(* Logix 5000 AddOnInstructionDefinition export AMCI_MA_SD_SMD_Linear_Follower_CIPSYNC; software revision 20.05 *)

TYPE AMCI_Motion_Axis_Output_Data :
STRUCT
   Control_Word_0 : INT;
   Control_Word_1 : INT;
   Position_or_Distance : DINT;
   Programmed_Speed : DINT;
   Acceleration : INT;
   Deceleration : INT;
   Output_Word_8 : INT;
   Output_Word_9 : INT;
END_STRUCT
END_TYPE

TYPE AMCI_Motion_Axis_Input_Data :
STRUCT
   Moving_CW : BOOL;
   Moving_CCW : BOOL;
   In_Hold_State : BOOL;
   Stopped : BOOL;
   At_Home : BOOL;
   Accelerating : BOOL;
   Decelerating : BOOL;
   Move_Complete : BOOL;
   Status_Word_0_Bit_8 : BOOL;
   Status_Word_0_Bit_9 : BOOL;
   Position_Invalid : BOOL;
   Input_Error : BOOL;
   Command_Error : BOOL;
   Configuration_Error : BOOL;
   Module_OK : BOOL;
   Mode_Flag : BOOL;
   IN1_Active : BOOL;
   IN2_Active : BOOL;
   IN3_Active : BOOL;
   IN4_Active : BOOL;
   Status_Word_1_Bit_4 : BOOL;
   Status_Word_1_Bit_5 : BOOL;
   Connection_Was_Lost : BOOL;
   Driver_Fault : BOOL;
   Status_Word_1_Bit_8 : BOOL;
   Invalid_Jog_Change : BOOL;
   Status_Word_1_Bit_10 : BOOL;
   Heartbeat_Bit : BOOL;
   Status_Word_1_Bit_12 : BOOL;
   Status_Word_1_Bit_13 : BOOL;
   Stall_Detected : BOOL;
   Drive_Is_Enabled : BOOL;
   Motor_Position : DINT;
   Encoder_Position : DINT;
   Trapped_Encoder_Position : DINT;
   Input_Word_8 : INT;
   Input_Word_9 : INT;
END_STRUCT
END_TYPE

ADD_ON_INSTRUCTION AMCI_MA_SD_SMD_Linear_Follower_CIPSYNC   (* revision 1.0, vendor AMCI, ExecuteEnableInFalse *)
// Linear Axis Follower for SD and SMD devices.   Will not work with SV integrated servo devices.
// Revision note:
// 8/8/24.  Added timesync functionality to a previously existing AOI.  Also added logic to preset the motor position to the master axis position when the rung with the AOI becomes true, or if the master axis position changes when motion is not occurring.
// Help:
// MOTION AXIS SD & SMD LINEAR FOLLOWER
// These AOIs will only work with the SD and SMD motion devices.  The SV motion devices have their own follower AOIs.
// AXIS INPUT DATA:  Input data from AMCI motion device.   Uses the AMCI_Motion_Axis_Input_Data User Defined Data Type.
// AXIS OUTPUT DATA; Output data from the AOI to the AMCI motion device.   Uses the AMCI_Motion_Axis_Output_Data User Defined Data Type.
// FOLLOWER POSITION: REAL DATA TYPE position directly from the motion axis.
// FOLLOWER VELOCITY: REAL DATA TYPE velocity directly from the motion axis.
// ACCELERATION & DECELERATION: An actual value or an INT DATA TYPE.  Larger acceleration and
//                                                             deceleration values will cause the motion device to more quickly react
//                                                              changes in the source position and velocity values.
// PROPORTIONAL COEFFICIENT:  A value of 1 or 2 is recommended
// NETWORK DELAY: A value of zero, or 1 to the RPI time, will work in most applications.
// RPI_TIME: The RPI time used when adding the AMCI Motion device to the network.   8ms is the default.
//                    Used to control how long the preset motor command is sent to the device when the rung with the
//                    AOI transitions from false to true.
// TIMESYNC: The PLC's time value used to more closely synchronize the motion data from the PLC's master
//                     axis with the output of the AMCI motion device.
// EN (Enable) Set when rung is true, Reset when rung is false
// DN (Done) Set when command is sent to the motion device.  Reset when the rung is false.
// ER (Error) Set when a command or input error failed to clear.  Reset when the rung is false.
// IP (In Process) Set when follower command is active, even if motion is not occurring.   Reset when the rung
//                         goes false.
VAR_IN_OUT
   Axis_Input_Data : AMCI_Motion_Axis_Input_Data; {required}
   Axis_Output_Data : AMCI_Motion_Axis_Output_Data; {required}
END_VAR
VAR_INPUT
   Current_System_Time : DINT; {required}
   _0_for_Normal_1_for_Continuous : BOOL;
   Master_Axis_Position : REAL; {required}
   Master_Axis_Velocity : REAL; {required}
   Acceleration : INT; {required}
   Deceleration : INT; {required}
   Proportional_Coefficient : INT; {required}
   RPI_time_in_ms : DINT; {required}
END_VAR
VAR_OUTPUT
   EN : BOOL; {visible}
   ER : BOOL; {visible}
   DN : BOOL; {visible}
   IP : BOOL; {visible}
END_VAR
VAR
   command_data_block : INT[10];
        [0]   // Command Bits MSW
        [1]   // Command Bits LSW
        [2]   // Upper Target Position
        [3]   // Lower Target Position
        [4]   // Upper Programmed Speed
        [5]   // Lower Programmed Speed
   axis_follower_position : DINT;
   axis_follower_velocity : DINT;
   Preset_Motor_Position_timer_dynanic : TIMER; {access None}
   preset_one_shot : BOOL; {access None}
   RPI_div_1000 : REAL; {access None}
   difference_scan_position : DINT; {access None}
   last_scan_position : DINT; {access None}
   position_difference : DINT; {access None}
   position_last_scan_linear_SMD : DINT; {access None}
END_VAR

ROUTINE EnableInFalse   (* ladder *)
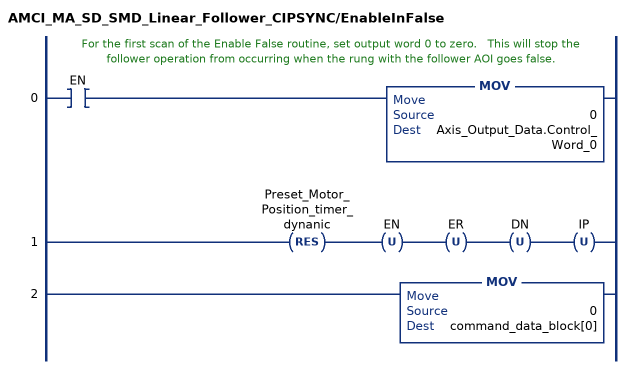
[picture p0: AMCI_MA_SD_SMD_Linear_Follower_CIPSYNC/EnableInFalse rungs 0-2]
   // For the first scan of the Enable False routine, set output word 0 to zero.   This will stop the follower operation from occurring when the rung with the follower AOI goes false.
   0: XIC(EN)MOV(0,Axis_Output_Data.Control_Word_0);
   1: RES(Preset_Motor_Position_timer_dynanic)OTU(EN)OTU(ER)OTU(DN)OTU(IP);
   2: MOV(0,command_data_block[0]);
END_ROUTINE

ROUTINE Logic   (* ladder *)
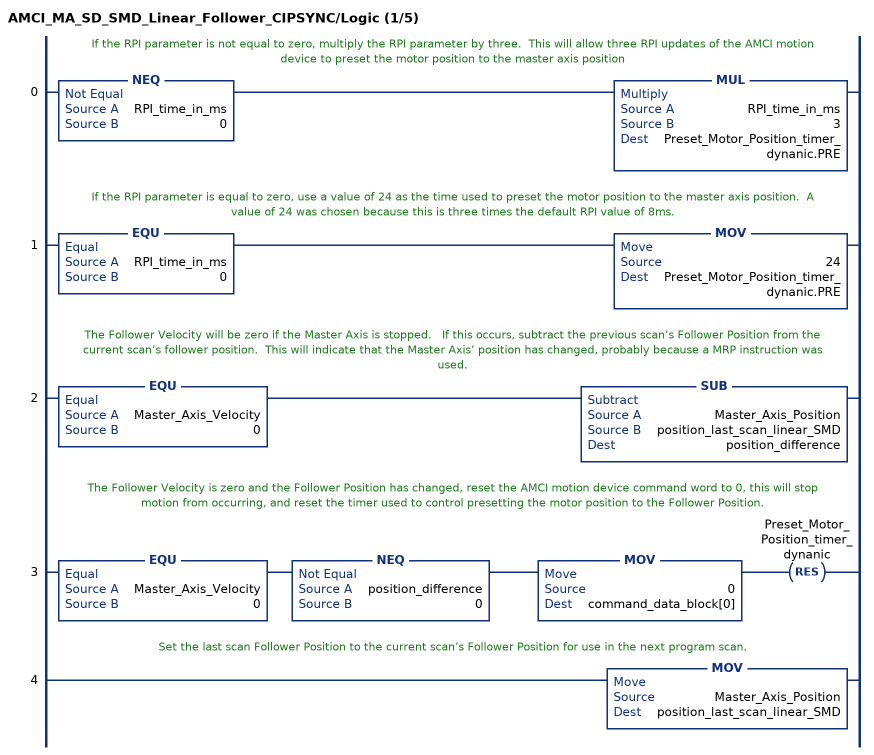
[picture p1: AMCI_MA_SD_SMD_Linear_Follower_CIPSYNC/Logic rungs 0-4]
   // If the RPI parameter is not equal to zero, multiply the RPI parameter by three.  This will allow three RPI updates of the AMCI motion device to preset the motor position to the master axis position
   0: NEQ(RPI_time_in_ms,0)MUL(RPI_time_in_ms,3,Preset_Motor_Position_timer_dynanic.PRE);
   // If the RPI parameter is equal to zero, use a value of 24 as the time used to preset the motor position to the master axis position.  A value of 24 was chosen because this is three times the default RPI value of 8ms.
   1: EQU(RPI_time_in_ms,0)MOV(24,Preset_Motor_Position_timer_dynanic.PRE);
   // The Follower Velocity will be zero if the Master Axis is stopped.   If this occurs, subtract the previous scan’s Follower Position from the current scan’s follower position.  This will indicate that the Master Axis’ position has changed, probably because a MRP instruction was used.
   2: EQU(Master_Axis_Velocity,0)SUB(Master_Axis_Position,position_last_scan_linear_SMD,position_difference);
   // The Follower Velocity is zero and the Follower Position has changed, reset the AMCI motion device command word to 0, this will stop motion from occurring, and reset the timer used to control presetting the motor position to the Follower Position.
   3: EQU(Master_Axis_Velocity,0)NEQ(position_difference,0)MOV(0,command_data_block[0])RES(Preset_Motor_Position_timer_dynanic);
   // Set the last scan Follower Position to the current scan’s Follower Position for use in the next program scan.
   4: MOV(Master_Axis_Position,position_last_scan_linear_SMD);
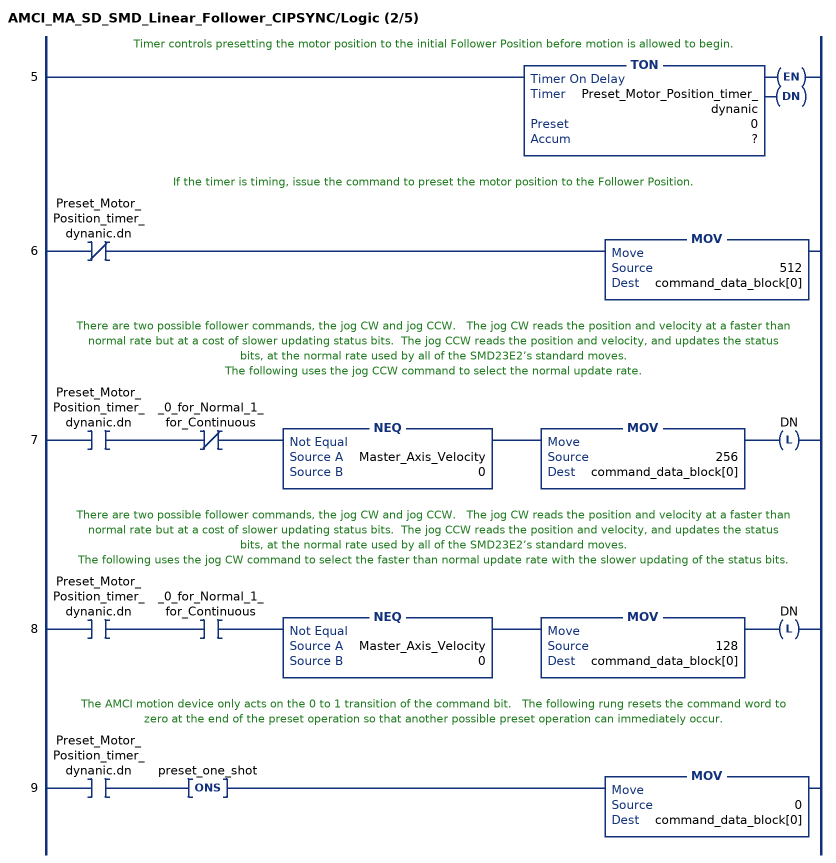
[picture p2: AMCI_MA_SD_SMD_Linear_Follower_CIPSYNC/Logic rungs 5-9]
   // Timer controls presetting the motor position to the initial Follower Position before motion is allowed to begin.
   5: TON(Preset_Motor_Position_timer_dynanic,?,?);
   // If the timer is timing, issue the command to preset the motor position to the Follower Position.
   6: XIO(Preset_Motor_Position_timer_dynanic.dn)MOV(512,command_data_block[0]);
   // There are two possible follower commands, the jog CW and jog CCW.   The jog CW reads the position and velocity at a faster than normal rate but at a cost of slower updating status bits.  The jog CCW reads the position and velocity, and updates the status bits, at the normal rate used by all of the SMD23E2’s standard moves.
   // The following uses the jog CCW command to select the normal update rate.
   7: XIC(Preset_Motor_Position_timer_dynanic.dn)XIO(_0_for_Normal_1_for_Continuous)NEQ(Master_Axis_Velocity,0)MOV(256,command_data_block[0])OTL(DN);
   // There are two possible follower commands, the jog CW and jog CCW.   The jog CW reads the position and velocity at a faster than normal rate but at a cost of slower updating status bits.  The jog CCW reads the position and velocity, and updates the status bits, at the normal rate used by all of the SMD23E2’s standard moves.
   // The following uses the jog CW command to select the faster than normal update rate with the slower updating of the status bits.
   8: XIC(Preset_Motor_Position_timer_dynanic.dn)XIC(_0_for_Normal_1_for_Continuous)NEQ(Master_Axis_Velocity,0)MOV(128,command_data_block[0])OTL(DN);
   // The AMCI motion device only acts on the 0 to 1 transition of the command bit.   The following rung resets the command word to zero at the end of the preset operation so that another possible preset operation can immediately occur.
   9: XIC(Preset_Motor_Position_timer_dynanic.dn)ONS(preset_one_shot)MOV(0,command_data_block[0]);
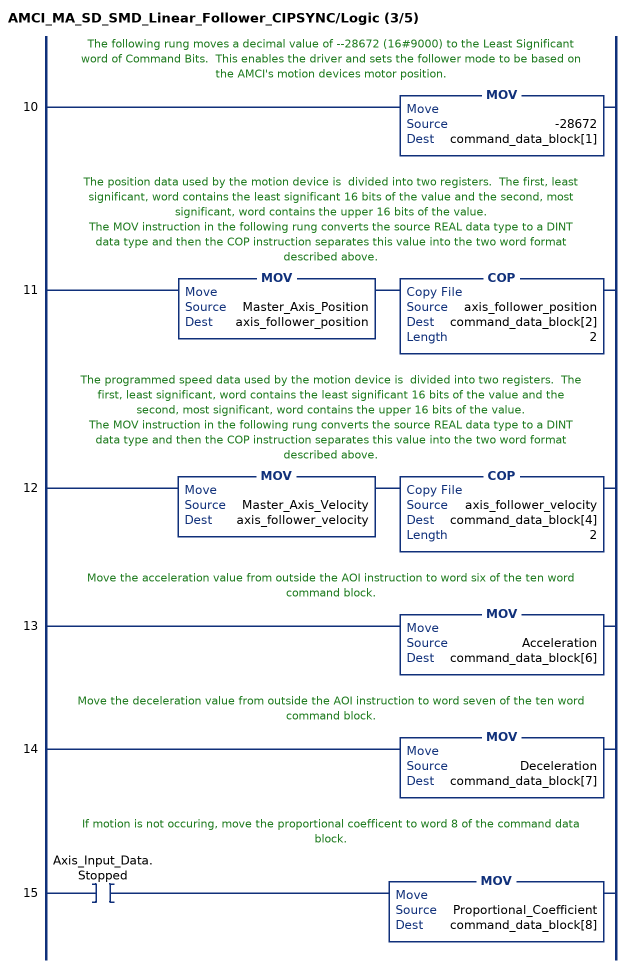
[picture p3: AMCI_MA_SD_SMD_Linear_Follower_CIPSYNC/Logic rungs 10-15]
   // The following rung moves a decimal value of --28672 (16#9000) to the Least Significant word of Command Bits.  This enables the driver and sets the follower mode to be based on the AMCI's motion devices motor position.
   10: MOV(-28672,command_data_block[1]);
   // The position data used by the motion device is  divided into two registers.  The first, least significant, word contains the least significant 16 bits of the value and the second, most significant, word contains the upper 16 bits of the value.
   // The MOV instruction in the following rung converts the source REAL data type to a DINT data type and then the COP instruction separates this value into the two word format described above.
   11: MOV(Master_Axis_Position,axis_follower_position)COP(axis_follower_position,command_data_block[2],2);
   // The programmed speed data used by the motion device is  divided into two registers.  The first, least significant, word contains the least significant 16 bits of the value and the second, most significant, word contains the upper 16 bits of the value.
   // The MOV instruction in the following rung converts the source REAL data type to a DINT data type and then the COP instruction separates this value into the two word format described above.
   12: MOV(Master_Axis_Velocity,axis_follower_velocity)COP(axis_follower_velocity,command_data_block[4],2);
   // Move the acceleration value from outside the AOI instruction to word six of the ten word command block.
   13: MOV(Acceleration,command_data_block[6]);
   // Move the deceleration value from outside the AOI instruction to word seven of the ten word command block.
   14: MOV(Deceleration,command_data_block[7]);
   // If motion is not occuring, move the proportional coefficent to word 8 of the command data block.
   15: XIC(Axis_Input_Data.Stopped)MOV(Proportional_Coefficient,command_data_block[8]);
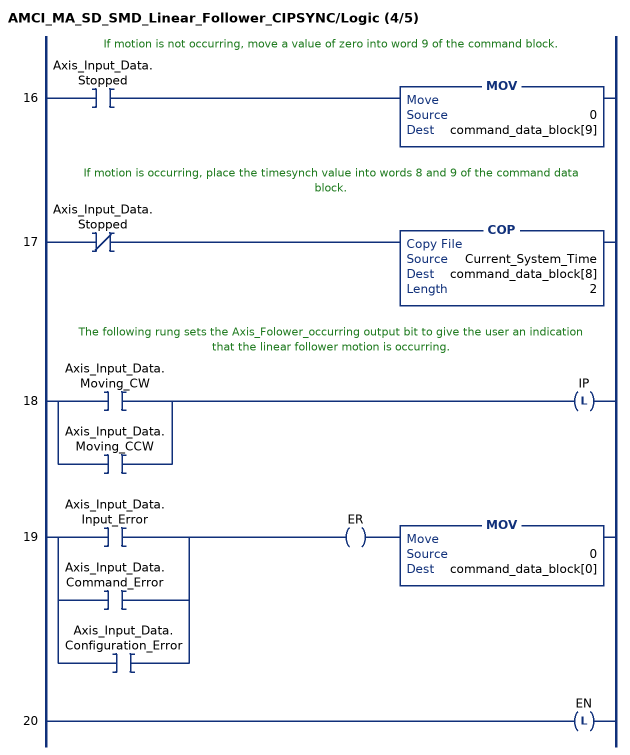
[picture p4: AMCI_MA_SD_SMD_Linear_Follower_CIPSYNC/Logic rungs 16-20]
   // If motion is not occurring, move a value of zero into word 9 of the command block.
   16: XIC(Axis_Input_Data.Stopped)MOV(0,command_data_block[9]);
   // If motion is occurring, place the timesynch value into words 8 and 9 of the command data block.
   17: XIO(Axis_Input_Data.Stopped)COP(Current_System_Time,command_data_block[8],2);
   // The following rung sets the Axis_Folower_occurring output bit to give the user an indication that the linear follower motion is occurring.
   18: [XIC(Axis_Input_Data.Moving_CW) ,XIC(Axis_Input_Data.Moving_CCW) ]OTL(IP);
   19: [XIC(Axis_Input_Data.Input_Error) ,XIC(Axis_Input_Data.Command_Error) ,XIC(Axis_Input_Data.Configuration_Error) ]OTE(ER)MOV(0,command_data_block[0]);
   20: OTL(EN);
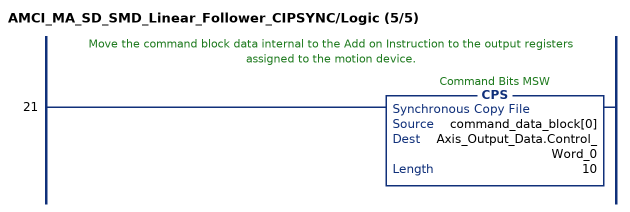
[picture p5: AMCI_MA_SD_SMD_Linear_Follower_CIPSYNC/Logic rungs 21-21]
   // Move the command block data internal to the Add on Instruction to the output registers assigned to the motion device.
   21: CPS(command_data_block[0],Axis_Output_Data.Control_Word_0,10);
END_ROUTINE
END_ADD_ON_INSTRUCTION
